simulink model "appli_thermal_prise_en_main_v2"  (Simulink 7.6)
settings: Solver=ode15s  StartTime=0.0  StopTime=120  RelTol=1e-3
StopFcn:
  | close all
  | load temp.mat
  | plot(x(1,:),x(2,:),x(1,:),x(3,:))
  | title('Transfert par convection')
  | %axis([0 9e5 298.12 298.16])
  | xlabel('temps')
  | grid
libraries: fl_lib x9, nesl_utility x4

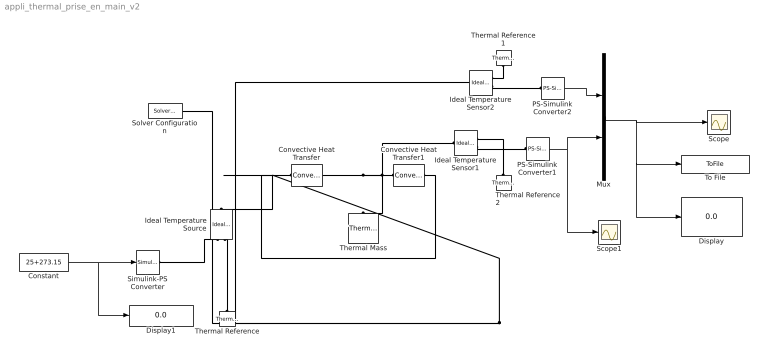
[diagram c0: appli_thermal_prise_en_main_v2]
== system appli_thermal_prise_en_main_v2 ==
  Constant : Constant  Value=25+273.15
  Convective Heat Transfer : fl_lib/Thermal/Thermal Elements/Convective Heat Transfer  DialogController=NetworkEngine.DynNeDlgSource  SystemSampleTime=-1  area=1 m^2  heat_tr_coeff=20 W/(m^2 * K)  Q_Log=off  T_Log=off  LocalVarNames=|Q|T  LocalVarDescs=|Q|T  LocalVarLogging=[0 0]
  Convective Heat Transfer1 : fl_lib/Thermal/Thermal Elements/Convective Heat Transfer  DialogController=NetworkEngine.DynNeDlgSource  SystemSampleTime=-1  area=1 m^2  heat_tr_coeff=20 W/(m^2 * K)  Q_Log=off  T_Log=off  LocalVarNames=|Q|T  LocalVarDescs=|Q|T  LocalVarLogging=[0 0]
  Display : Display
  Display1 : Display
  Ideal Temperature Sensor1 : fl_lib/Thermal/Thermal Sensors/Ideal Temperature Sensor  DialogController=NetworkEngine.DynNeDlgSource  SystemSampleTime=-1  Qs_Log=off  Ts_Log=off  LocalVarNames=|Qs|Ts  LocalVarDescs=|Qs|Ts  LocalVarLogging=[0 0]
  Ideal Temperature Sensor2 : fl_lib/Thermal/Thermal Sensors/Ideal Temperature Sensor  DialogController=NetworkEngine.DynNeDlgSource  SystemSampleTime=-1  Qs_Log=off  Ts_Log=off  LocalVarNames=|Qs|Ts  LocalVarDescs=|Qs|Ts  LocalVarLogging=[0 0]
  Ideal Temperature Source : fl_lib/Thermal/Thermal Sources/Ideal Temperature Source  DialogController=NetworkEngine.DynNeDlgSource  SystemSampleTime=-1  Q_Log=off  T_Log=off  LocalVarNames=|Q|T  LocalVarDescs=|Q|T  LocalVarLogging=[0 0]
  Mux : Mux  Inputs=2
  PS-Simulink Converter1 : nesl_utility/PS-Simulink Converter  DialogController=NetworkEngine.DynNeUtilDlgSource  SystemSampleTime=-1  PhysicalDomain=network_engine_domain  LeftPortType=input  RightPortType=output  SubClassName=ps_output  Unit=1  AffineConversion=off
  PS-Simulink Converter2 : nesl_utility/PS-Simulink Converter  DialogController=NetworkEngine.DynNeUtilDlgSource  SystemSampleTime=-1  PhysicalDomain=network_engine_domain  LeftPortType=input  RightPortType=output  SubClassName=ps_output  Unit=1  AffineConversion=off
  Scope : Scope
  Scope1 : Scope
  Simulink-PS Converter : nesl_utility/Simulink-PS Converter  DialogController=NetworkEngine.DynNeUtilDlgSource  SystemSampleTime=-1  PhysicalDomain=network_engine_domain  LeftPortType=input  RightPortType=output  SubClassName=ps_input  Unit=1  AffineConversion=off  InputFilterTimeConstant=.001  UdotUserProvided=0
  Solver Configuration : nesl_utility/Solver Configuration  DialogController=NetworkEngine.DynNeUtilDlgSource  SystemSampleTime=-1  PhysicalDomain=network_engine_domain  LeftPortType=input  RightPortType=generic  SubClassName=solver  Accelerate=off  Profile=off  ResidualTolerance=1e-9  MaxNonlinIter=12  MaxModeIter=2  DoFixedCost=off  UseLocalSampling=off  DoDC=on  LinearAlgebra=Full  LocalSolverSampleTime=.001  LocalSolverChoice=NE_BACKWARD_EULER_ADVANCER  UseLocalSolver=off
  Thermal Mass : fl_lib/Thermal/Thermal Elements/Thermal Mass  DialogController=NetworkEngine.DynNeDlgSource  SystemSampleTime=-1  mass=1 kg  sp_heat=447 J/kg/K  init_temp=0 C  Q_Log=off  LocalVarNames=|Q  LocalVarDescs=|Q  LocalVarLogging=0
  Thermal Reference : fl_lib/Thermal/Thermal Elements/Thermal Reference  DialogController=NetworkEngine.DynNeDlgSource  SystemSampleTime=-1  Q_Log=off  LocalVarNames=|Q  LocalVarDescs=|Q  LocalVarLogging=0
  Thermal Reference1 : fl_lib/Thermal/Thermal Elements/Thermal Reference  DialogController=NetworkEngine.DynNeDlgSource  SystemSampleTime=-1  Q_Log=off  LocalVarNames=|Q  LocalVarDescs=|Q  LocalVarLogging=0
  Thermal Reference2 : fl_lib/Thermal/Thermal Elements/Thermal Reference  DialogController=NetworkEngine.DynNeDlgSource  SystemSampleTime=-1  Q_Log=off  LocalVarNames=|Q  LocalVarDescs=|Q  LocalVarLogging=0
  To File : ToFile  Filename=temp.mat  MatrixName=x
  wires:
  Constant/1 -> Simulink-PS Converter/1, Display1/1
  Mux/1 -> Scope/1, To File/1, Display/1
  PS-Simulink Converter2/1 -> Mux/1
  PS-Simulink Converter1/1 -> Mux/2, Scope1/1
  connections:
  Ideal Temperature Sensor1/RConn2 -- PS-Simulink Converter1/LConn1
  Thermal Reference2/LConn1 -- Ideal Temperature Sensor1/RConn1
  Simulink-PS Converter/RConn1 -- Ideal Temperature Source/RConn1
  Thermal Reference/LConn1 -- Ideal Temperature Source/RConn2
  Convective Heat Transfer1/LConn1 -- Thermal Mass/LConn1 -- Ideal Temperature Sensor1/LConn1 -- Convective Heat Transfer/RConn1
  Thermal Reference1/LConn1 -- Ideal Temperature Sensor2/RConn1
  Ideal Temperature Sensor2/RConn2 -- PS-Simulink Converter2/LConn1
  Convective Heat Transfer1/RConn1 -- Ideal Temperature Source/LConn1 -- Ideal Temperature Sensor2/LConn1 -- Solver Configuration/RConn1 -- Convective Heat Transfer/LConn1
